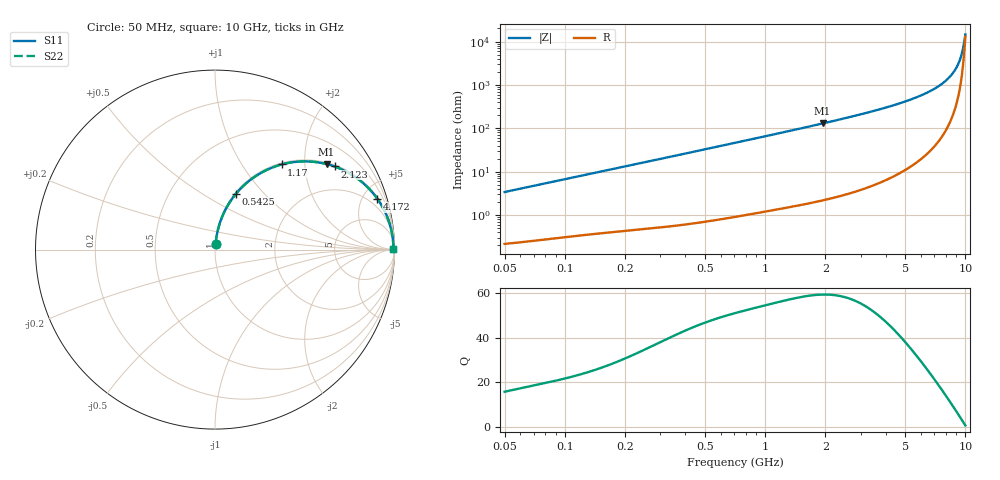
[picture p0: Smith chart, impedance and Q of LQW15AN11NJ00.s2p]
!Murata Part Number: LQW15AN11NJ00
!These Parameters are Measured in Series Mode Connection
!  o--[Z]--o
!Port1  Port2
!  o-------o
!Freq. Start=50[MHz] Stop=10[GHz], 401[Steps]
# Hz S RI R 50
!Freq.(Hz)	S 11(Real)	S 11(Imag)	S 21(Real)	S 21(Imag)	S 12(Real)	S 12(Imag)	S 22(Real)	S 22(Imag)
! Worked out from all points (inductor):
!   401 points, 50 MHz to 10 GHz, reference 50 ohm
!   read as one part in series: L = 10.7 nH near 51.34 MHz
!   highest Q = 59.5 at 1.935 GHz (marker M1), where L = 10.6 nH
!   S11 on the Smith chart (normalised r, x): 50 MHz: 1.00, +0.07; 542.5 MHz: 1.01, +0.71; 1.17 GHz: 1.03, +1.53; 2.123 GHz: 1.05, +2.84; 4.172 GHz: 1.14, +6.34; 10 GHz: open
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5e7  0.00328 0.0336  0.9967 -0.0336  0.9967 -0.0336  0.00328 0.0336
1.214486e8  0.00977 0.0795  0.9902 -0.0795  0.9902 -0.0795  0.00977 0.0795
2.949953e8  0.0405 0.1843  0.9595 -0.1843  0.9595 -0.1843  0.0405 0.1843
5.425422e8  0.1163 0.3104  0.8837 -0.3104  0.8837 -0.3104  0.1163 0.3104
7.071068e8  0.18 0.3745  0.82 -0.3745  0.82 -0.3745  0.18 0.3745
9.094607e8  0.2642 0.4317  0.7358 -0.4317  0.7358 -0.4317  0.2642 0.4317
1.169723e9  0.3713 0.4743  0.6287 -0.4743  0.6287 -0.4743  0.3713 0.4743
1.717543e9  0.5623 0.4877  0.4377 -0.4877  0.4377 -0.4877  0.5623 0.4877
1.934999e9  0.622 0.4766  0.378 -0.4766  0.378 -0.4766  0.622 0.4766
2.122994e9  0.6666 0.4631  0.3334 -0.4631  0.3334 -0.4631  0.6666 0.4631
2.99582e9  0.8096 0.3837  0.1904 -0.3837  0.1904 -0.3837  0.8096 0.3837
4.171863e9  0.9044 0.2833  0.0956 -0.2833  0.0956 -0.2833  0.9044 0.2833
5.156693e9  0.9444 0.2159  0.0556 -0.2159  0.0556 -0.2159  0.9444 0.2159
6.207365e9  0.9686 0.1574  0.0314 -0.1574  0.0314 -0.1574  0.9686 0.1574
7.181012e9  0.9816 0.1118  0.0184 -0.1118  0.0184 -0.1118  0.9816 0.1118
7.983737e9  0.9881 0.0784  0.0119 -0.0784  0.0119 -0.0784  0.9881 0.0784
8.644138e9  0.9915 0.053  0.00853 -0.053  0.00853 -0.053  0.9915 0.053
9.114482e9  0.993 0.0355  0.00704 -0.0355  0.00704 -0.0355  0.993 0.0355
9.359165e9  0.9935 0.0265  0.00653 -0.0265  0.00653 -0.0265  0.9935 0.0265
9.48396e9  0.9937 0.022  0.00634 -0.022  0.00634 -0.022  0.9937 0.022
9.868415e9  0.994 0.00798  0.00604 -0.00798  0.00604 -0.00798  0.994 0.00798
1e10  0.994 0.00316  0.00605 -0.00316  0.00605 -0.00316  0.994 0.00316
